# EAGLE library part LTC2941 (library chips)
I2C Battery Gas Gauge with External Sense Resistor
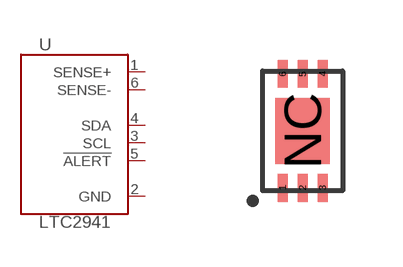
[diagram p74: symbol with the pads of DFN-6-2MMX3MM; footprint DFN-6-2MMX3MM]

Designator prefix U

## LTC2941 (DIGIKEY: LTC2941IDCB#TRMPBFCT-ND)  [DFN-6-2MMX3MM]
1  SENSE+  oc
2  GND  oc
3  SCL  oc
4  SDA  oc
5  !ALERT  oc
6  SENSE-  oc

## Footprint DFN-6-2MMX3MM (pad centres in mm)
smd 0.25 x 0.7: 1 -0.5,-1.425; 2 0,-1.425; 3 0.5,-1.425; 4 0.5,1.425; 5 0,1.425; 6 -0.5,1.425
smd 1.35 x 1.65: NC 0,0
